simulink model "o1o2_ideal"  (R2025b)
settings: Solver=VariableStepAuto  StartTime=0.0  StopTime=50.0  RelTol=1e-3
undefined symbols (not defined in the file): D, F, I, kp_pi, P, Ti_pi
libraries: slpidlib x2

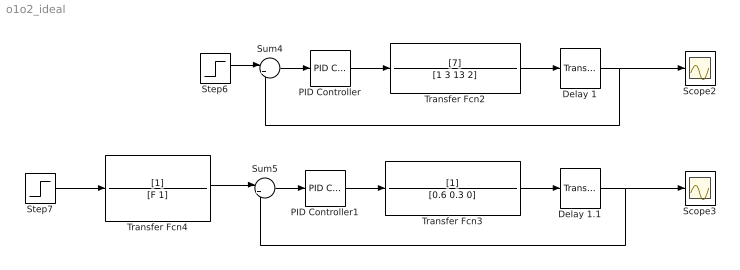
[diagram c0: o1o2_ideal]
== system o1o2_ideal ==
  Delay 1 : TransportDelay  DelayTime=2
  Delay 1.1 : TransportDelay  DelayTime=1.5
  PID Controller : slpidlib/PID Controller  Controller=PI  Form=Ideal  TimeDomain=Continuous-time  UseExternalTs=off  SampleTime=-1  IntegratorMethod=Forward Euler  FilterMethod=Forward Euler  ControllerParametersSource=internal  P=kp_pi*0.36  I=1/Ti_pi  UseKiTs=off  D=0  UseExternalDerivativeSource=off  N=100  UseFilter=on  TunerSelectOption=Transfer Function Based (PID Tuner App)  InitialConditionSource=internal  InitialConditionForIntegrator=0  InitialConditionForFilter=0  DifferentiatorICPrevScaledInput=0  ExternalReset=none  TrackingMode=off  Kt=1  LimitOutput=off  SatLimitsSource=internal  UpperSaturationLimit=inf  LowerSaturationLimit=-inf  LinearizeAsGain=on  AntiWindupMode=none  Kb=1  LimitIntegrator=off  UpperIntegratorSaturationLimit=inf  LowerIntegratorSaturationLimit=-inf  POutMin=[]  POutMax=[]  IOutMin=[]  IOutMax=[]  DOutMin=[]  DOutMax=[]  NOutMin=[]  NOutMax=[]  SumOutMin=[]  SumOutMax=[]  SaturationOutMin=[]  SaturationOutMax=[]  PParamMin=[]  PParamMax=[]  IParamMin=[]  IParamMax=[]  DParamMin=[]  DParamMax=[]  NParamMin=[]  NParamMax=[]  KbParamMin=[]  KbParamMax=[]  KtParamMin=[]  KtParamMax=[]  KbOutMin=[]  KbOutMax=[]  KtOutMin=[]  KtOutMax=[]  IntegratorOutMin=[]  IntegratorOutMax=[]  FilterOutMin=[]  FilterOutMax=[]  SumI1OutMin=[]  SumI1OutMax=[]  SumI2OutMin=[]  SumI2OutMax=[]  SumI3OutMin=[]  SumI3OutMax=[]  SumI4OutMin=[]  SumI4OutMax=[]  SumDOutMin=[]  SumDOutMax=[]  DifferentiatorOutMin=[]  DifferentiatorOutMax=[]  FilterDiffOutCoefMin=[]  FilterDiffOutCoefMax=[]  ReciprocalOutMin=[]  ReciprocalOutMax=[]  SumDenOutMin=[]  SumDenOutMax=[]  SumNumOutMin=[]  SumNumOutMax=[]  DivideOutMin=[]  DivideOutMax=[]  UdiffTsProdOutMin=[]  UdiffTsProdOutMax=[]  NTsProdOutMin=[]  NTsProdOutMax=[]  UintegralTsProdOutMin=[]  UintegralTsProdOutMax=[]  UngainTsProdOutMin=[]  UngainTsProdOutMax=[]  ClampingZeroOutDataTypeStr=Inherit: Inherit via back propagation  ClampingZeroOutMin=[]  ClampingZeroOutMax=[]  FilterDenConstantOutDataTypeStr=Inherit: Inherit via back propagation  FilterDenConstantOutMin=[]  FilterDenConstantOutMax=[]  PCopyOutDataTypeStr=Inherit: Inherit via back propagation  PCopyOutMin=[]  PCopyOutMax=[]  NCopyOutDataTypeStr=Inherit: Inherit via back propagation  NCopyOutMin=[]  NCopyOutMax=[]  IntegratorContinuousStateAttributes=''  IntegratorStateMustResolveToSignalObject=off  IntegratorRTWStateStorageClass=Auto  FilterContinuousStateAttributes=''  FilterStateMustResolveToSignalObject=off  FilterRTWStateStorageClass=Auto  ParallelPVariant=Passthrough  IdealPVariant=InternalParameters  IVariant=InternalParameters  DVariant=Disabled  IntegratorVariant=Continuous  SatVariant=Disabled  AWVariant=Passthrough  PCopyVariant=Disabled  TRVariant=Disabled  FdbkBlocksVariant=Forward  IdealPFdbkVariant=Disabled  SatFdbkVariant=Disabled  DerivativeFilterVariant=Disabled  NVariant=Disabled  NCopyVariant=Disabled_SignalSpec  FilterICVariant=Disabled  IntegratorICVariant=InternalICs  ExternalResetVariant=Disabled  TRSumVariant=Passthrough  SumFdbkVariant=Disabled  SumVariant=Sum_PI  TsampFilterVariant=InternalTs  TsampNgainVariant=Passthrough  TsampIntegralVariant=Disabled_SignalSpec  ExternalSaturationOutDataTypeStr=Inherit: Same as second input  DerivativeSourceVariant=Disabled  PreIntVariant=InternalPreInt
  PID Controller1 : slpidlib/PID Controller  Controller=PID  Form=Parallel  TimeDomain=Continuous-time  UseExternalTs=off  SampleTime=-1  IntegratorMethod=Forward Euler  FilterMethod=Forward Euler  ControllerParametersSource=internal  P=P  I=I  UseKiTs=off  D=D  UseExternalDerivativeSource=off  N=100  UseFilter=on  TunerSelectOption=Transfer Function Based (PID Tuner App)  InitialConditionSource=internal  InitialConditionForIntegrator=0  InitialConditionForFilter=0  DifferentiatorICPrevScaledInput=0  ExternalReset=none  TrackingMode=off  Kt=1  LimitOutput=off  SatLimitsSource=internal  UpperSaturationLimit=inf  LowerSaturationLimit=-inf  LinearizeAsGain=on  AntiWindupMode=none  Kb=1  LimitIntegrator=off  UpperIntegratorSaturationLimit=inf  LowerIntegratorSaturationLimit=-inf  POutMin=[]  POutMax=[]  IOutMin=[]  IOutMax=[]  DOutMin=[]  DOutMax=[]  NOutMin=[]  NOutMax=[]  SumOutMin=[]  SumOutMax=[]  SaturationOutMin=[]  SaturationOutMax=[]  PParamMin=[]  PParamMax=[]  IParamMin=[]  IParamMax=[]  DParamMin=[]  DParamMax=[]  NParamMin=[]  NParamMax=[]  KbParamMin=[]  KbParamMax=[]  KtParamMin=[]  KtParamMax=[]  KbOutMin=[]  KbOutMax=[]  KtOutMin=[]  KtOutMax=[]  IntegratorOutMin=[]  IntegratorOutMax=[]  FilterOutMin=[]  FilterOutMax=[]  SumI1OutMin=[]  SumI1OutMax=[]  SumI2OutMin=[]  SumI2OutMax=[]  SumI3OutMin=[]  SumI3OutMax=[]  SumI4OutMin=[]  SumI4OutMax=[]  SumDOutMin=[]  SumDOutMax=[]  DifferentiatorOutMin=[]  DifferentiatorOutMax=[]  FilterDiffOutCoefMin=[]  FilterDiffOutCoefMax=[]  ReciprocalOutMin=[]  ReciprocalOutMax=[]  SumDenOutMin=[]  SumDenOutMax=[]  SumNumOutMin=[]  SumNumOutMax=[]  DivideOutMin=[]  DivideOutMax=[]  UdiffTsProdOutMin=[]  UdiffTsProdOutMax=[]  NTsProdOutMin=[]  NTsProdOutMax=[]  UintegralTsProdOutMin=[]  UintegralTsProdOutMax=[]  UngainTsProdOutMin=[]  UngainTsProdOutMax=[]  ClampingZeroOutDataTypeStr=Inherit: Inherit via back propagation  ClampingZeroOutMin=[]  ClampingZeroOutMax=[]  FilterDenConstantOutDataTypeStr=Inherit: Inherit via back propagation  FilterDenConstantOutMin=[]  FilterDenConstantOutMax=[]  PCopyOutDataTypeStr=Inherit: Inherit via back propagation  PCopyOutMin=[]  PCopyOutMax=[]  NCopyOutDataTypeStr=Inherit: Inherit via back propagation  NCopyOutMin=[]  NCopyOutMax=[]  IntegratorContinuousStateAttributes=''  IntegratorStateMustResolveToSignalObject=off  IntegratorRTWStateStorageClass=Auto  FilterContinuousStateAttributes=''  FilterStateMustResolveToSignalObject=off  FilterRTWStateStorageClass=Auto  ParallelPVariant=InternalParameters  IdealPVariant=Disabled  IVariant=InternalParameters  DVariant=InternalParameters  IntegratorVariant=Continuous  SatVariant=Disabled  AWVariant=Passthrough  PCopyVariant=Disabled  TRVariant=Disabled  FdbkBlocksVariant=Forward  IdealPFdbkVariant=Disabled  SatFdbkVariant=Disabled  DerivativeFilterVariant=ContFilter  NVariant=InternalParameters  NCopyVariant=Disabled  FilterICVariant=InternalICsFilter  IntegratorICVariant=InternalICs  ExternalResetVariant=Disabled  TRSumVariant=Passthrough  SumFdbkVariant=Disabled  SumVariant=Sum_PID  TsampFilterVariant=InternalTs  TsampNgainVariant=Passthrough  TsampIntegralVariant=Disabled_SignalSpec  ExternalSaturationOutDataTypeStr=Inherit: Same as second input  DerivativeSourceVariant=ErrorSignal  PreIntVariant=InternalPreInt
  Scope2 : Scope
  Scope3 : Scope
  Step6 : Step  Time=0  After=0.3  SampleTime=0
  Step7 : Step  Time=0  After=0.3  SampleTime=0
  Sum4 : Sum  Inputs=|+-
  Sum5 : Sum  Inputs=|+-
  Transfer Fcn2 : TransferFcn  Numerator=[7]  Denominator=[1 3 13 2]
  Transfer Fcn3 : TransferFcn  Denominator=[0.6 0.3 0]
  Transfer Fcn4 : TransferFcn  Denominator=[F 1]
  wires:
  PID Controller1/1 -> Transfer Fcn3/1
  Delay 1.1/1 -> Sum5/2, Scope3/1
  Transfer Fcn4/1 -> Sum5/1
  Step7/1 -> Transfer Fcn4/1
  PID Controller/1 -> Transfer Fcn2/1
  Sum4/1 -> PID Controller/1
  Sum5/1 -> PID Controller1/1
  Step6/1 -> Sum4/1
  Transfer Fcn2/1 -> Delay 1/1
  Transfer Fcn3/1 -> Delay 1.1/1
  Delay 1/1 -> Scope2/1, Sum4/2
